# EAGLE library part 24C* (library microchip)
Serial EEPROM 1 K/2 K/4 K
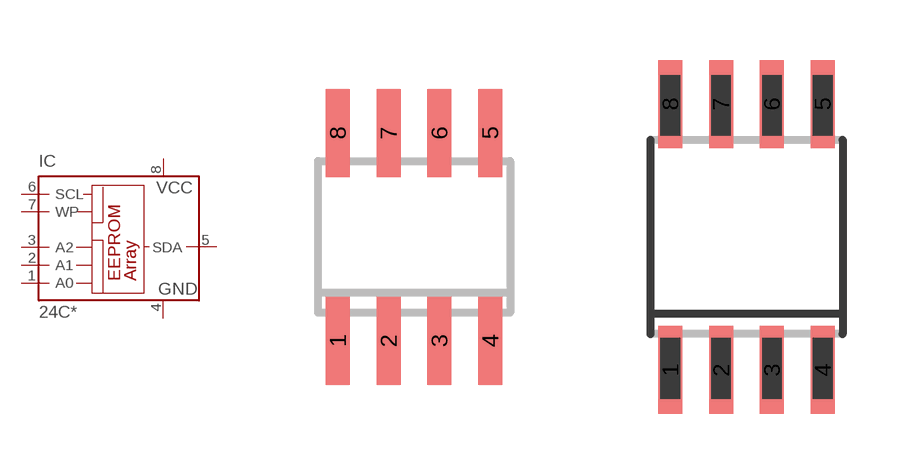
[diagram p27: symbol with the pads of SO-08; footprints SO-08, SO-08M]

Designator prefix IC

## 24C01SN (MPN: CAT24C01WI-GT3; OC_FARNELL: 1718117; OC_NEWARK: 06R0487), 24C01ASN (MPN: AT24C01BN-SH-B; OC_FARNELL: 1362638; OC_NEWARK: 50M3313), 24C01CSN (MF: MICROCHIP; MPN: 24C01C/SN; OC_FARNELL: unknown; OC_NEWARK: 96K4061), 24C02SN (OC_FARNELL: unknown; OC_NEWARK: unknown), 24C02ASN (OC_FARNELL: unknown; OC_NEWARK: unknown), 24C02CSN (MF: MICROCHIP; MPN: 24C02C/SN; OC_FARNELL: 1607552; OC_NEWARK: 96K4065), 24C04SN (MPN: M24C04-WMN6P; OC_FARNELL: 9882812; OC_NEWARK: 83K1376), 24C04ASN (OC_FARNELL: unknown; OC_NEWARK: unknown), 24C04CSN (OC_FARNELL: unknown; OC_NEWARK: unknown)  [SO-08]
1  A0  in
2  A1  in
3  A2  in
4  GND  pwr
5  SDA
6  SCL  in
7  WP  in
8  VCC  pwr

## 24C01SM (MPN: M24C01-WMN6P; OC_FARNELL: 9882790; OC_NEWARK: 24M5068), 24C01ASM (MPN: AT24C01BN-SH-B; OC_FARNELL: 1362638; OC_NEWARK: 50M3313), 24C01CSM (MPN: M24C01-WMN6P; OC_FARNELL: 9882790; OC_NEWARK: 24M5068), 24C02SM (MF: MICROCHIP; MPN: 24C02C-I/SN; OC_FARNELL: 1084339; OC_NEWARK: 96K4063), 24C02ASM (MPN: M24C02-WMN6P; OC_FARNELL: 9882804; OC_NEWARK: 10M9771), 24C02CSM (MF: MICROCHIP; MPN: 24C02C-I/SN; OC_FARNELL: 1084339; OC_NEWARK: 96K4063), 24C04SM (MPN: CAT24C04WI-G; OC_FARNELL: 1631136; OC_NEWARK: 06R0507), 24C04ASM (MPN: AT24C04BN-SH-B; OC_FARNELL: 1362643; OC_NEWARK: 50M3316)  [SO-08M]
Pads as for SO-08

## 24C01P (MF: MICROCHIP; MPN: 24C01C-I/P; OC_FARNELL: 1847800; OC_NEWARK: 92C6948), 24C01AP (MF: Arrow Electronics; MPN: M24C01-WBN6P; OC_FARNELL: 9882782; OC_NEWARK: 93K7306), 24C01CP (MF: MICROCHIP; MPN: 24C01C/P; OC_FARNELL: 3662901; OC_NEWARK: 96K4060), 24C02P (OC_FARNELL: unknown; OC_NEWARK: unknown), 24C02AP (MPN: M24C02-WBN6P; OC_FARNELL: 1094256; OC_NEWARK: 11M0888), 24C02CP (MF: MICROCHIP; MPN: 24C02C/P; OC_FARNELL: 1296567; OC_NEWARK: 96K4064), 24C04P (MPN: M24C04-WBN6P; OC_FARNELL: 1094258; OC_NEWARK: 02M5802), 24C04AP (MPN: AT24C04B-PU; OC_FARNELL: 1362642; OC_NEWARK: 50M3315), 24C04CP (MPN: CAT24C04LI-G; OC_FARNELL: 1718374; OC_NEWARK: 73P4460)  [DIL8]
Pads as for SO-08

## 24C01SL (OC_FARNELL: unknown; OC_NEWARK: unknown), 24C02SL (OC_FARNELL: unknown; OC_NEWARK: unknown), 24C04SL (OC_FARNELL: unknown; OC_NEWARK: unknown)  [SO-14]
2  A0  in
3  A1  in
5  A2  in
6  GND  pwr
9  SDA
10  SCL  in
12  WP  in
13  VCC  pwr

## Footprint SO-08 (pad centres in mm)
Small Outline Narrow Plastic Gull Wing 150-mil body, package type SN
smd 0.6 x 2.2: 1 -1.905,-2.6; 2 -0.635,-2.6; 3 0.635,-2.6; 4 1.905,-2.6; 5 1.905,2.6; 6 0.635,2.6; 7 -0.635,2.6; 8 -1.905,2.6

## Footprint SO-08M (pad centres in mm)
Small Outline Medium Plastic Gull Wing 207-mil body, package type SM
smd 0.6 x 2.2: 1 -1.905,-3.33; 2 -0.635,-3.33; 3 0.635,-3.33; 4 1.905,-3.33; 5 1.905,3.33; 6 0.635,3.33; 7 -0.635,3.33; 8 -1.905,3.33

## Footprint DIL8 (pad centres in mm)
Dual In Line package type P
drill 0.813 long: 1 -3.81,-3.81; 2 -1.27,-3.81; 3 1.27,-3.81; 4 3.81,-3.81; 5 3.81,3.81; 6 1.27,3.81; 7 -1.27,3.81; 8 -3.81,3.81

## Footprint SO-14 (pad centres in mm)
Small Outline Narrow Plastic Gull Wing 150-mil body, package type SL
smd 0.6 x 2.2: 1 -3.81,-2.6; 2 -2.54,-2.6; 3 -1.27,-2.6; 4 0,-2.6; 5 1.27,-2.6; 6 2.54,-2.6; 7 3.81,-2.6; 8 3.81,2.6; 9 2.54,2.6; 10 1.27,2.6; 11 0,2.6; 12 -1.27,2.6; 13 -2.54,2.6; 14 -3.81,2.6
